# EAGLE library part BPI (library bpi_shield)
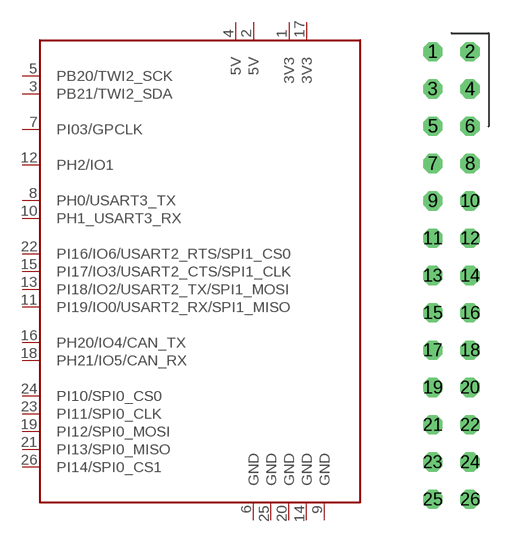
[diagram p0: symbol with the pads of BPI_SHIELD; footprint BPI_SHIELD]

Designator prefix -

## BPI  [BPI_SHIELD]
1  3V3
2  5V
3  PB21/TWI2_SDA
4  5V
5  PB20/TWI2_SCK
6  GND
7  PI03/GPCLK
8  PH0/USART3_TX
9  GND
10  PH1_USART3_RX
11  PI19/IO0/USART2_RX/SPI1_MISO
12  PH2/IO1
13  PI18/IO2/USART2_TX/SPI1_MOSI
14  GND
15  PI17/IO3/USART2_CTS/SPI1_CLK
16  PH20/IO4/CAN_TX
17  3V3
18  PH21/IO5/CAN_RX
19  PI12/SPI0_MOSI
20  GND
21  PI13/SPI0_MISO
22  PI16/IO6/USART2_RTS/SPI1_CS0
23  PI11/SPI0_CLK
24  PI10/SPI0_CS0
25  GND
26  PI14/SPI0_CS1

## Footprint BPI_SHIELD (pad centres in mm)
drill 0.8 octagon: 1 0,0; 2 2.54,0; 3 0,-2.54; 4 2.54,-2.54; 5 0,-5.08; 6 2.54,-5.08; 7 0,-7.62; 8 2.54,-7.62; 9 0,-10.16; 10 2.54,-10.16; 11 0,-12.7; 12 2.54,-12.7; 13 0,-15.24; 14 2.54,-15.24; 15 0,-17.78; 16 2.54,-17.78; 17 0,-20.32; 18 2.54,-20.32; 19 0,-22.86; 20 2.54,-22.86; 21 0,-25.4; 22 2.54,-25.4; 23 0,-27.94; 24 2.54,-27.94; 25 0,-30.48; 26 2.54,-30.48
